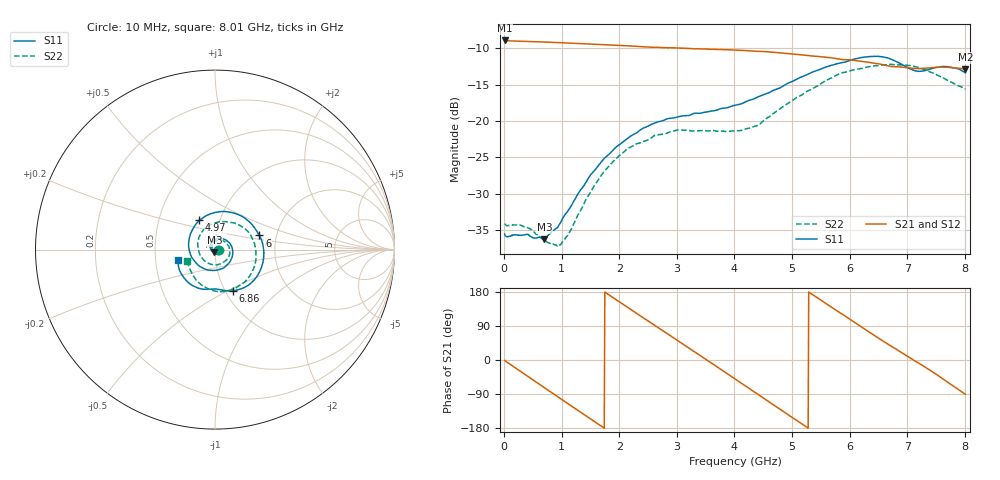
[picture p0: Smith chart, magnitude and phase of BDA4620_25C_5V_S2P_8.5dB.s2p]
!Agilent Technologies,E5071B,MY42404982,A.09.10
!Date: Wed May 06 08:59:55 2026
!Data & Calibration Information:
!Freq	S11:SOLT2(ON)	S21:SOLT2(ON)	S12:SOLT2(ON)	S22:SOLT2(ON)
# Hz S RI R 50
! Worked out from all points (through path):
!   801 points, 10 MHz to 8.01 GHz, reference 50 ohm
!   highest |S21| = -8.94 dB at 10 MHz (marker M1); lowest = -12.9 dB at 8.01 GHz (marker M2)
!   group delay of S21, straight-line fit = 281 ps
!   lowest |S11| = -36.3 dB at 700 MHz (marker M3), VSWR 1.03, Z = 49.7 - j1.49 ohm
!   |S11| at or under -10 dB: start of sweep to end of sweep
!   |S22| runs from -37.2 to -12.2 dB; largest |S21 - S12| = 0.0015
!   S11 on the Smith chart (normalised r, x): 10 MHz: 1.03, -0.00; 4.97 GHz: 0.80, +0.27; 6 GHz: 1.63, +0.27; 6.86 GHz: 1.08, -0.53; 8.01 GHz: 0.65, -0.08
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1e7  0.0166 -0.0012  0.357 -0.0076  0.3576 -0.00799  0.0195 -0.00121
3.3e8  0.0126 -0.0105  0.2898 -0.2  0.29 -0.201  0.0163 -0.00951
7e8  -0.00294 -0.015  0.1017 -0.3331  0.102 -0.3337  0.00252 -0.015
9.8e8  -0.0189 -0.00648  -0.071 -0.3374  -0.0713 -0.3379  -0.0114 -0.00828
1.35e9  -0.0261 0.0224  -0.2601 -0.2186  -0.2602 -0.2188  -0.0195 0.0157
1.65e9  -0.0103 0.0489  -0.3304 -0.0549  -0.3311 -0.055  -0.00936 0.0388
1.94e9  0.0213 0.0622  -0.3107 0.1137  -0.3112 0.1141  0.0157 0.0527
2.32e9  0.0697 0.0465  -0.1679 0.2782  -0.1685 0.2786  0.0553 0.0429
2.68e9  0.0987 -0.0019  0.0278 0.3188  0.0282 0.3192  0.0796 0.00968
3e9  0.0886 -0.0582  0.1924 0.2524  0.1927 0.2525  0.0802 -0.0317
3.39e9  0.0336 -0.1077  0.3042 0.072  0.3048 0.0716  0.0427 -0.0739
3.69e9  -0.0289 -0.1148  0.296 -0.0913  0.2962 -0.092  -0.00462 -0.0848
4.01e9  -0.0964 -0.0843  0.1975 -0.2346  0.1975 -0.2352  -0.058 -0.0628
4.48e9  -0.1474 0.0281  -0.0415 -0.2972  -0.0417 -0.2977  -0.096 0.0223
4.97e9  -0.0864 0.1629  -0.2457 -0.1523  -0.2463 -0.1524  -0.0416 0.1286
5.35e9  0.0396 0.2121  -0.2775 0.0327  -0.2778 0.0327  0.0584 0.1551
6e9  0.2477 0.0786  -0.0817 0.25  -0.0819 0.2504  0.2162 0.044
6.34e9  0.2662 -0.0746  0.0704 0.2421  0.071 0.2422  0.2258 -0.066
6.68e9  0.1727 -0.2067  0.1817 0.1538  0.1825 0.1543  0.1747 -0.1709
6.86e9  0.0991 -0.2298  0.2153 0.0943  0.216 0.0942  0.1255 -0.2078
7.43e9  -0.0597 -0.2212  0.2002 -0.1171  0.2006 -0.1173  -0.0634 -0.2051
8.01e9  -0.2058 -0.0573  -0.00134 -0.2266  -0.00116 -0.2272  -0.1537 -0.0608
